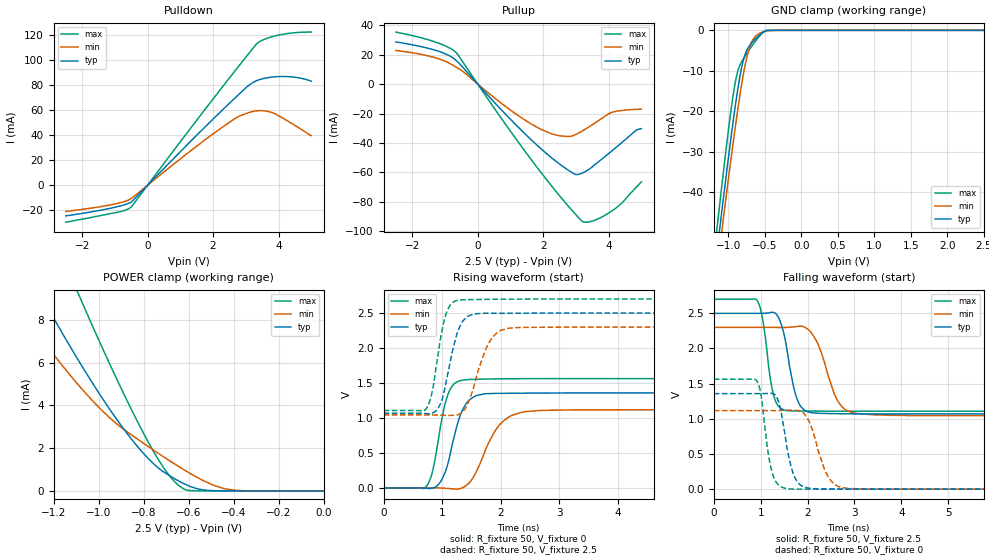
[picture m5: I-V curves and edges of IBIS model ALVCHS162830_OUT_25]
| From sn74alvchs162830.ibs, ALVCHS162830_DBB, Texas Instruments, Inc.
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[Model]   ALVCHS162830_OUT_25
Model_type  3-state
Enable   Active-Low
Vref =   0.0
Rref =   500
Cref =   30p
Vmeas =   1.25
| variable   typ   min   max
C_comp   4.09pF   2.69pF   6.19pF
| C_pullup   3.72pF   2.81pF   5.86pF
| C_pulldown   3.11pF   2.69pF   3.82pF
| C_tri-state   5.45pF   4.59pF   6.19pF
[Temperature Range]   40   100   -40
| Ambient temperature   25   85   -40
[Voltage range]   2.5   2.3   2.7
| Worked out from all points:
|   slope of the pulldown table from 0 to 0.375 V, typ, clamps not added: 37 ohm
|   slope of the pullup table from 0 to 0.375 V, typ, clamps not added: 40.7 ohm
|   GND clamp passes 1 mA (typ) near -0.56 V on its own axis
|   POWER clamp passes 1 mA (typ) near -0.72 V on its own axis
|   rising waveform, R_fixture 50, V_fixture 0: 20-80 % time 262ps typ, 395ps min, 209ps max; typ from 0 V to 1.36 V
|   falling waveform, R_fixture 50, V_fixture 2.5: 20-80 % time 248ps typ, 380ps min, 193ps max; typ from 2.5 V to 1.07 V
|   rising waveform, R_fixture 50, V_fixture 2.5: 20-80 % time 230ps typ, 300ps min, 190ps max; typ from 1.07 V to 2.5 V
|   falling waveform, R_fixture 50, V_fixture 0: 20-80 % time 231ps typ, 326ps min, 190ps max; typ from 1.36 V to 0 V
[GND Clamp]
| ALVCHS162830_OUT_25
|   Voltage   I(typ)   I(min)   I(max)
-2.5V     -271.8mA   -269.3mA   -276.7mA
-1.17V    -56.83mA   -61.33mA   -51.14mA
-1.135V   -51.49mA   -56.16mA   -45.51mA
-1.105V   -46.96mA   -51.77mA   -40.74mA
-1.075V   -42.47mA   -47.42mA   -36.03mA
-920mV    -20.59mA   -25.85mA   -14.34mA
-870mV    -14.46mA   -19.46mA   -10.05mA
-810mV    -8.529mA   -12.5mA    -7.505mA
-700mV    -3.539mA   -3.676mA   -4.442mA
-565mV    -1.014mA   -660.1uA   -1.262mA
-450mV    -10.66uA   -124.4uA   -6.278uA
2.5V      56.77pA    96.6nA     5.744pA
[POWER Clamp]
| ALVCHS162830_OUT_25
|   Voltage   I(typ)   I(min)   I(max)
-2.5V     36.17mA    28.44mA    48.49mA
-1.39V    11.75mA    9.132mA    16.87mA
-1.265V   9.314mA    7.293mA    13.61mA
-1.24V    8.841mA    6.94mA     12.97mA
-1.095V   6.207mA    5.026mA    9.354mA
-1.075V   5.86mA     4.782mA    8.869mA
-825mV    2.055mA    2.412mA    3.206mA
-715mV    922.2uA    1.624mA    1.157mA
-640mV    442.5uA    1.117mA    225.5uA
-545mV    67.38uA    541.2uA    2.747uA
-415mV    738.9nA    60.96uA    15.44nA
-31.15fV  56.77pA    368.2pA    6.49pA
[Pulldown]
| ALVCHS162830_OUT_25
|   Voltage   I(typ)   I(min)   I(max)
-2.5V     -24.5mA    -20.96mA   -29.54mA
-1.095V   -18.19mA   -15.53mA   -22.48mA
-715mV    -15.7mA    -13.09mA   -20.2mA
-500mV    -13.39mA   -10.5mA    -17.31mA
2.045V    53.97mA    41.83mA    70.4mA
2.725V    71.03mA    54.11mA    93.15mA
3.115V    80.2mA     58.22mA    106mA
3.37V     83.9mA     59.54mA    113.8mA
3.695V    86.03mA    58.85mA    117.8mA
3.905V    86.66mA    56.92mA    119.4mA
4.385V    86.57mA    49.66mA    121.6mA
5V        83.08mA    39.59mA    122.3mA
[Pullup]
| ALVCHS162830_OUT_25
|   Voltage   I(typ)   I(min)   I(max)
-2.5V     28.66mA    22.84mA    35.35mA
-1.26V    22.76mA    17.67mA    28.33mA
-660mV    16.05mA    11.53mA    21.39mA
955mV     -22.91mA   -16.96mA   -30.63mA
1.905V    -43.38mA   -30.39mA   -59.26mA
2.715V    -57.76mA   -35.55mA   -81.57mA
2.99V     -61.45mA   -34.29mA   -88.53mA
3.195V    -60.47mA   -31.85mA   -93.31mA
3.535V    -55.58mA   -27.14mA   -92.87mA
4.075V    -45.86mA   -19.45mA   -86.6mA
4.83V     -31.59mA   -17.18mA   -70.47mA
5V        -30.25mA   -17mA      -66.48mA
[Ramp]
| ALVCHS162830_OUT_25
| variable   typ   min   max
dV/dt_r   0.82/2.71E-10   0.68/4.22E-10   0.94/2.20E-10
dV/dt_f   0.87/2.58E-10   0.77/3.98E-10   0.96/2.00E-10
R_load = 50
[Rising Waveform]
| ALVCHS162830_OUT_25
R_fixture =   50
C_fixture =   0
L_fixture =   0
V_fixture =   0
V_fixture_min = 0
V_fixture_max = 0
|   Time   V(typ)   V(min)   V(max)
0s        -3.799uV   -10.6uV    -1.15uV
705ps     -1.656mV   912.5uV    4.62mV
820ps     -4.481mV   1.368mV    189.7mV
920ps     35.98mV    874.5uV    615.7mV
1.135ns   480.1mV    -9.374mV   1.409V
1.31ns    1.041V     -8.581mV   1.534V
1.485ns   1.271V     96.5mV     1.551V
2.01ns    1.353V     930.1mV    1.56V
2.7ns     1.357V     1.109V     1.563V
49.99ns   1.358V     1.117V     1.563V
[Falling Waveform]
| ALVCHS162830_OUT_25
R_fixture =   50
C_fixture =   0
L_fixture =   0
V_fixture =   2.5
V_fixture_min = 2.3
V_fixture_max = 2.7
|   Time   V(typ)   V(min)   V(max)
0s        2.5V       2.3V       2.7V
920ps     2.499V     2.3V       2.688V
1.29ns    2.51V      2.299V     1.304V
1.48ns    2.254V     2.299V     1.133V
1.67ns    1.562V     2.305V     1.111V
1.845ns   1.186V     2.318V     1.11V
2.135ns   1.083V     2.171V     1.11V
2.745ns   1.072V     1.166V     1.108V
3.445ns   1.069V     1.057V     1.108V
49.99ns   1.069V     1.046V     1.108V
[Rising Waveform]
| ALVCHS162830_OUT_25
R_fixture =   50
C_fixture =   0
L_fixture =   0
V_fixture =   2.5
V_fixture_min = 2.3
V_fixture_max = 2.7
|   Time   V(typ)   V(min)   V(max)
0s        1.069V     1.046V     1.108V
705ps     1.065V     1.045V     1.115V
815ps     1.066V     1.044V     1.324V
900ps     1.105V     1.042V     1.75V
1.085ns   1.592V     1.037V     2.531V
1.245ns   2.183V     1.042V     2.679V
1.36ns    2.393V     1.099V     2.69V
1.83ns    2.497V     2.119V     2.697V
2.32ns    2.498V     2.294V     2.7V
49.99ns   2.5V       2.3V       2.7V
[Falling Waveform]
| ALVCHS162830_OUT_25
R_fixture =   50
C_fixture =   0
L_fixture =   0
V_fixture =   0
V_fixture_min = 0
V_fixture_max = 0
|   Time   V(typ)   V(min)   V(max)
0s        1.358V     1.117V     1.563V
905ps     1.358V     1.117V     1.555V
1ns       1.359V     1.117V     1.368V
1.26ns    1.361V     1.117V     205.3mV
1.405ns   1.191V     1.118V     47.07mV
1.665ns   283.2mV    1.123V     907.5uV
2.02ns    14.41mV    980.8mV    241.4uV
2.51ns    1.348mV    112mV      318.3uV
3.02ns    218.8uV    5.425mV    -16.62uV
49.99ns   -3.826uV   -10.14uV   -1.16uV
